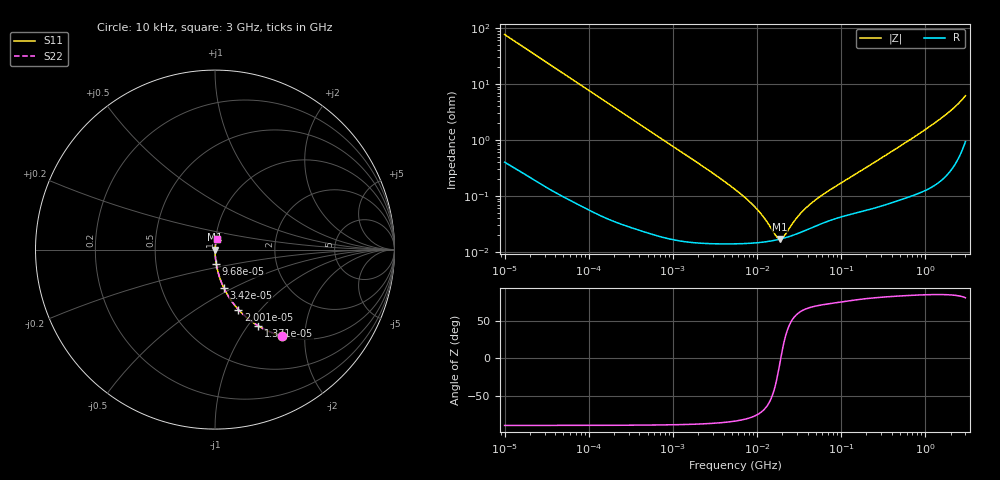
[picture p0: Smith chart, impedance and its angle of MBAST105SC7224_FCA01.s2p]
! MBAST105SC7224_FCA01  S-PARAMETER MODEL  ( Standard Model )
! Model Generated by TAIYO YUDEN Corporation (http://www.ty-top.com)
! Version 2.0
! TAIYO YUDEN Control No. 240621
! Copyright(c) 2023 TAIYO YUDEN CO.,LTD. All Rights Reserved.
! Product Description (link to TY-COMPAS)
! https://ds.yuden.co.jp/TYCOMPAS/or/detail?pn=MBAST105SC7224KFCA01&u=M
! Products Name : Multilayer Ceramic Capacitors
! Characteristics :
!  Capacitance : 0.22 [uF] , Rated Voltage : 25 [V] , TCC : X7S
!  Case Size : 1.0 x 0.5 / 0.039 x 0.02 [mm/inch] , Thickness : 0.5 / 0.02 [mm/inch]
!  (Conditions: Temperature = 25 [degC] , DC Bias Voltage = 0 [V])
! External Node Assignments :
!  1  o---| |---o  2
! GND o---------o GND
! Frequency Range : 10kHz  -  3GHz  [ 401 STEP ]
# MHZ S RI R 50
! Freq[MHz].  S11 Real  S11 Imag  S21 Real  S21 Imag  S12 Real  S12 Imag  S22 Real  S22 Imag
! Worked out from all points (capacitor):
!   401 points, 10 kHz to 3 GHz, reference 50 ohm
!   read as one part in series: C = 207 nF near 10.65 kHz
!   lowest |Z| = 17.1 mohm at 18.73 MHz (marker M1)
!   series resonance near 19.15 MHz, so ESL is about 330 pH
!   S11 on the Smith chart (normalised r, x): 10 kHz: 1.01, -1.54; 13.71 kHz: 1.01, -1.12; 20.01 kHz: 1.00, -0.77; 34.2 kHz: 1.00, -0.45; 96.8 kHz: 1.00, -0.16; 3 GHz: 1.02, +0.12
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0.01  0.3721 -0.4807  0.6279 0.4807  0.6279 0.4807  0.3721 -0.4807
0.013707  0.2408 -0.4249  0.7592 0.4249  0.7592 0.4249  0.2408 -0.4249
0.02001  0.1305 -0.3341  0.8695 0.3341  0.8695 0.3341  0.1305 -0.3341
0.034199  0.0496 -0.2142  0.9504 0.2142  0.9504 0.2142  0.0496 -0.2142
0.082683  0.00933 -0.0927  0.9907 0.0927  0.9907 0.0927  0.00933 -0.0927
0.096801  0.00693 -0.0794  0.9931 0.0794  0.9931 0.0794  0.00693 -0.0794
0.219733  0.00158 -0.0353  0.9984 0.0353  0.9984 0.0353  0.00158 -0.0353
0.683653  0.000321 -0.0114  0.9997 0.0114  0.9997 0.0114  0.000321 -0.0114
2.652321  0.00015 -0.00289  0.9999 0.00289  0.9999 0.00289  0.00015 -0.00289
5.477226  0.000142 -0.00131  0.9999 0.00131  0.9999 0.00131  0.000142 -0.00131
9.97066  0.000147 -0.000568  0.9999 0.000568  0.9999 0.000568  0.000147 -0.000568
12.43293  0.000152 -0.00036  0.9998 0.00036  0.9998 0.00036  0.000152 -0.00036
16.51234  0.000163 -0.000119  0.9998 0.000119  0.9998 0.000119  0.000163 -0.000119
18.73182  0.00017 -1.77e-05  0.9998 1.77e-05  0.9998 1.77e-05  0.00017 -1.77e-05
20.5901  0.000176 5.75e-05  0.9998 -5.75e-05  0.9998 -5.75e-05  0.000176 5.75e-05
31.02164  0.000216 0.000386  0.9998 -0.000386  0.9998 -0.000386  0.000216 0.000386
45.28751  0.000274 0.000716  0.9997 -0.000716  0.9997 -0.000716  0.000274 0.000716
72.67256  0.000365 0.00122  0.9996 -0.00122  0.9996 -0.00122  0.000365 0.00122
374.4521  0.000768 0.00583  0.9992 -0.00583  0.9992 -0.00583  0.000768 0.00583
1452.736  0.00227 0.0228  0.9977 -0.0228  0.9977 -0.0228  0.00227 0.0228
2120.803  0.00444 0.0356  0.9956 -0.0356  0.9956 -0.0356  0.00444 0.0356
3000  0.0129 0.0599  0.9871 -0.0599  0.9871 -0.0599  0.0129 0.0599
